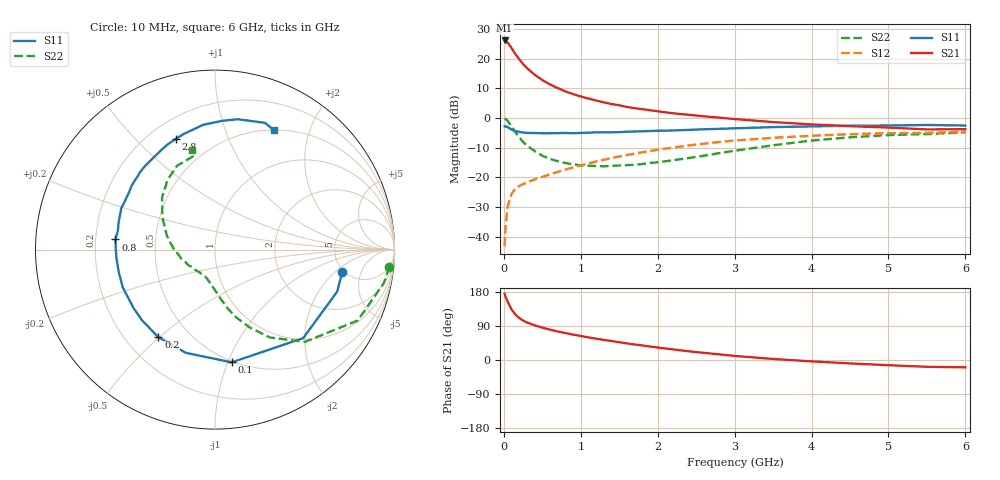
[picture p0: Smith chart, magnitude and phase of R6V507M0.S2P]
! SIEMENS Small Signal Semiconductors
! BFR193
! Si NPN RF Bipolar Junction Transistor in SOT23
! VCE = 0.5 V  IC = 7 mA
! Common Emitter S-Parameters:  May  1996
# GHz  S  MA  R  50
!  f  S11  S21  S12  S22
! GHz  MAG  ANG  MAG  ANG  MAG  ANG  MAG  ANG
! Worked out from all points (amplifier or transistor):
!   36 points, 10 MHz to 6 GHz, reference 50 ohm
!   highest |S21| = 26.1 dB at 10 MHz (marker M1)
!   |S21| within 3 dB of that: start of sweep to 111 MHz
!   unconditionally stable (mu >= 1): 757.2 MHz to 2.491 GHz; 5.899 GHz to end of sweep
!   at 250 MHz: K = 0.55, MSG = 20.2 dB, |S12| = -22.3 dB
!   at 1.4 GHz: K = 1.08, MAG = 7.4 dB, |S12| = -13.5 dB
!   at 6 GHz: K = 1.00, MAG = 0.3 dB, |S12| = -4.6 dB
!   S11 on the Smith chart (normalised r, x): 10 MHz: 4.85, -2.47; 100 MHz: 0.49, -1.03; 200 MHz: 0.34, -0.50; 800 MHz: 0.28, +0.05; 2.8 GHz: 0.31, +0.66; 6 GHz: 0.51, +1.50
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0.01  0.7202 -9.8  20.14 174.6  0.0069 85.2  0.9761 -5.6
0.02  0.7197 -19.0  19.72 168.7  0.0135 80.7  0.9591 -11.2
0.05  0.6961 -45.1  18.43 153.4  0.0323 68.5  0.8881 -26.4
0.1  0.6349 -81.6  15.02 133.5  0.0525 55.8  0.7175 -45.8
0.15  0.5976 -105.8  11.87 120.0  0.0645 48.6  0.5763 -58.1
0.2  0.581 -122.9  9.724 110.9  0.0713 45.4  0.4724 -66.2
0.25  0.5661 -135.8  8.083 104.1  0.0768 44.1  0.3945 -72.7
0.3  0.5586 -144.3  6.889 99.2  0.0818 44.4  0.3435 -77.1
0.4  0.5554 -157.7  5.348 91.7  0.0919 45.5  0.276 -83.4
0.5  0.5506 -167.0  4.333 85.5  0.1012 47.4  0.2307 -89.3
0.6  0.5513 -174.9  3.658 80.1  0.1122 49.2  0.2032 -94.5
0.8  0.5574 174.2  2.796 71.2  0.1347 51.2  0.1739 -103.0
0.9  0.5513 168.9  2.515 67.1  0.1469 51.9  0.1644 -106.9
1.1  0.5627 160.4  2.117 59.7  0.1715 52.6  0.1567 -116.5
1.3  0.5696 152.7  1.826 53.1  0.1973 52.1  0.153 -125.7
1.6  0.5852 142.6  1.529 43.8  0.2366 50.3  0.1601 -138.8
2.2  0.6132 125.5  1.195 28.0  0.3166 44.3  0.1933 -164.2
2.8  0.654 109.5  1.01 15.0  0.3929 35.8  0.2551 170.2
3.5  0.6985 95.4  0.85 2.8  0.462 24.7  0.3454 148.2
4.5  0.7377 80.0  0.725 -9.0  0.5318 10.1  0.4709 124.0
5.5  0.759 68.5  0.639 -17.9  0.5569 -3.6  0.5332 103.4
6  0.7421 63.5  0.645 -19.4  0.5882 -7.7  0.572 103.1
